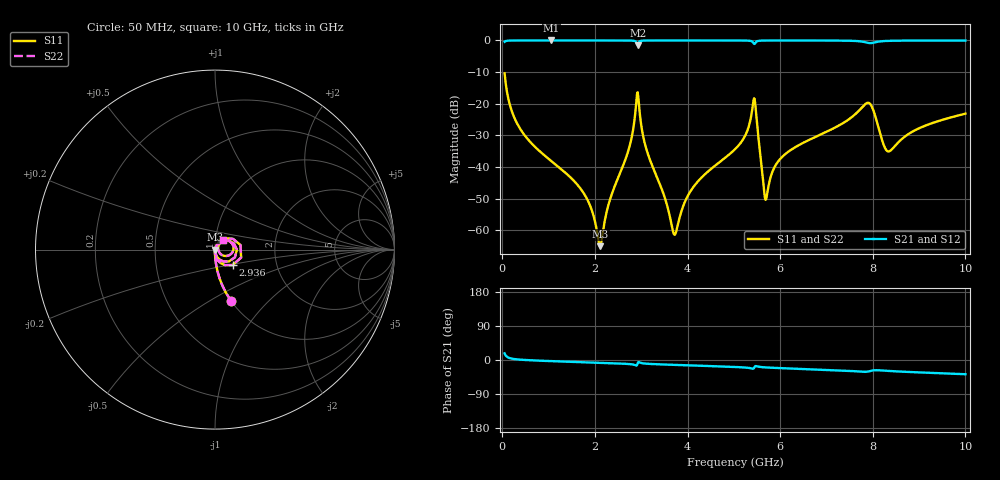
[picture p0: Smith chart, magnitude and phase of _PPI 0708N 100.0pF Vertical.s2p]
! S-Parameter data specifications (vertical orientation):
! Substrate: 40-mil Rogers 3003C, Substrate thickness, H=1.016mm, Dielectric constant, Er=3, Conductor thickness, T_mtl=0.043mm, Loss Tangent, Tand=0.003
! PCB Mounting Pad Footprint: Pad width, PadW=2.54mm , Pad length, PadL=0.51mm , Pad gap, PadG (edge-to-edge)=0.71mm , Reference planes=1.73mm apart
! Created Tue Jan 16 08:54:40 2018
# GHz S MA R 50
! 2 Port Network Data from SP1.SP block
! freq  magS11  angS11  magS21  angS21  magS12  angS12  magS22  angS22
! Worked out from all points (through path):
!   801 points, 50 MHz to 10 GHz, reference 50 ohm
!   highest |S21| = 0.00 dB at 1.057 GHz (marker M1); lowest = -1.4 dB at 2.923 GHz (marker M2)
!   group delay of S21, straight-line fit = 10.8 ps
!   lowest |S11| = -65.0 dB at 2.115 GHz (marker M3), VSWR 1.00, Z = 50.1 - j0.00451 ohm
!   |S11| at or under -10 dB: start of sweep to end of sweep
!   |S22| runs from -65.0 to -10.4 dB; largest |S21 - S12| = 0
!   S11 on the Smith chart (normalised r, x): 50 MHz: 1.00, -0.63; 2.936 GHz: 1.20, -0.21; 10 GHz: 1.09, +0.12
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0.05  0.3025 -72.5  0.9529 17.4  0.9529 17.4  0.3025 -72.5
0.3485  0.04475 -88.4  0.9988 1.3  0.9988 1.3  0.04475 -88.4
1.057438  0.01249 -91.4  0.9995 -3.0  0.9995 -3.0  0.01249 -91.4
1.716625  0.004297 -89.5  0.9995 -5.7  0.9995 -5.7  0.004297 -89.5
2.114625  0.0005652 -4.6  0.9993 -7.4  0.9993 -7.4  0.0005652 -4.6
2.326062  0.003083 69.0  0.9992 -8.3  0.9992 -8.3  0.003083 69.0
2.7365  0.01987 71.3  0.9969 -10.7  0.9969 -10.7  0.01987 71.3
2.923062  0.1522 -17.1  0.849 -8.9  0.849 -8.9  0.1522 -17.1
2.9355  0.1303 -41.4  0.891 -5.9  0.891 -5.9  0.1303 -41.4
3.08475  0.02252 -89.6  0.9958 -9.5  0.9958 -9.5  0.02252 -89.6
3.370812  0.006138 -90.8  0.9987 -11.4  0.9987 -11.4  0.006138 -90.8
3.7315  0.0008656 -2.7  0.999 -13.0  0.999 -13.0  0.0008656 -2.7
4.117063  0.004748 65.4  0.999 -14.5  0.999 -14.5  0.004748 65.4
5.025  0.01917 67.3  0.9982 -18.4  0.9982 -18.4  0.01917 67.3
5.261312  0.03332 62.9  0.9951 -20.0  0.9951 -20.0  0.03332 62.9
5.435437  0.1219 -0.2  0.885 -21.2  0.885 -21.2  0.1219 -0.2
5.696625  0.003125 5.3  0.9969 -19.7  0.9969 -19.7  0.003125 5.3
5.982687  0.01299 62.0  0.9981 -21.3  0.9981 -21.3  0.01299 62.0
6.691625  0.02838 61.9  0.9975 -24.5  0.9975 -24.5  0.02838 61.9
7.898062  0.1039 7.4  0.9157 -30.5  0.9157 -30.5  0.1039 7.4
8.345812  0.01769 8.4  0.9855 -28.9  0.9855 -28.9  0.01769 8.4
10  0.06976 50.5  0.9948 -37.5  0.9948 -37.5  0.06976 50.5
